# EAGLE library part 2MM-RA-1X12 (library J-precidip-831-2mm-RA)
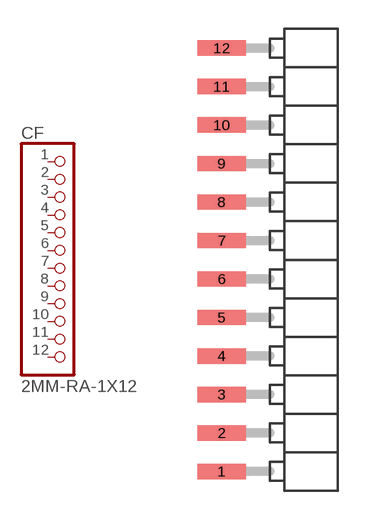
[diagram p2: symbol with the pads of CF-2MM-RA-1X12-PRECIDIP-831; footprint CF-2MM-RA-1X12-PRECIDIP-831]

Designator prefix CF

## 2MM-RA-1X12  [CF-2MM-RA-1X12-PRECIDIP-831]
1  1  pas
2  2  pas
3  3  pas
4  4  pas
5  5  pas
6  6  pas
7  7  pas
8  8  pas
9  9  pas
10  10  pas
11  11  pas
12  12  pas

## Footprint CF-2MM-RA-1X12-PRECIDIP-831 (pad centres in mm)
smd 2.5 x 0.8: 1 -3.25,-11; 2 -3.25,-9; 3 -3.25,-7; 4 -3.25,-5; 5 -3.25,-3; 6 -3.25,-1; 7 -3.25,1; 8 -3.25,3; 9 -3.25,5; 10 -3.25,7; 11 -3.25,9; 12 -3.25,11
